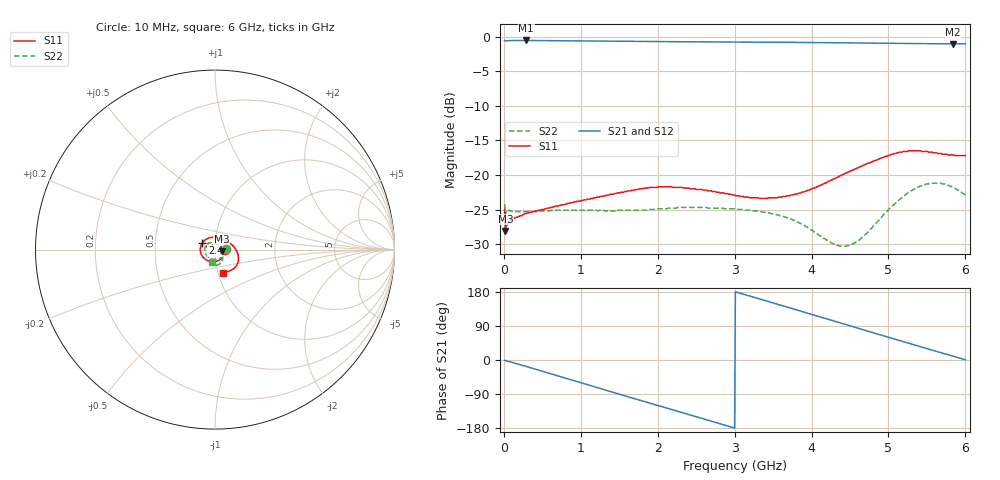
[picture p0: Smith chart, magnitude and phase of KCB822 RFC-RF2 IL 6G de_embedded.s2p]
!Agilent	"Technologies,N5230A,MY45001650,A.07.50.48"
!Agilent	N5230A:	A.07.50.48
!Date:	"Wednesday,"	February	"12,"	2014	15:18:42
!Correction:	S11(Full	2	"Port(1,2))"
!S21(Full	2	"Port(1,2))"
!S12(Full	2	"Port(1,2))"
!S22(Full	2	"Port(1,2))"
!S2P	File:	Measurements:	"S11,"	"S21,"	"S12,"	S22:
#	Hz	S	dB	R	50
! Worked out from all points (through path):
!   600 points, 10 MHz to 6 GHz, reference 50 ohm
!   highest |S21| = -0.55 dB at 290 MHz (marker M1); lowest = -1.0 dB at 5.84 GHz (marker M2)
!   group delay of S21, straight-line fit = 167 ps
!   lowest |S11| = -28.1 dB at 20 MHz (marker M3), VSWR 1.08, Z = 54 - j0.863 ohm
!   |S11| at or under -10 dB: start of sweep to end of sweep
!   |S22| runs from -30.3 to -21.2 dB; largest |S21 - S12| = 0.016
!   S11 on the Smith chart (normalised r, x): 10 MHz: 1.12, -0.00; 2.47 GHz: 0.87, +0.07; 6 GHz: 1.05, -0.28
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1e7  -25.00 -1.6  -0.55 -0.9  -0.55 -1.1  -24.20 3.1
2e7  -28.10 -11.7  -0.59 -1.4  -0.59 -1.4  -25.70 -4.1
5e7  -27.00 -6.7  -0.59 -3.4  -0.59 -3.4  -25.10 -4.4
2.9e8  -25.60 -18.8  -0.55 -16.9  -0.55 -17.0  -25.30 -13.0
6.4e8  -24.60 -46.1  -0.58 -38.2  -0.58 -38.2  -25.10 -33.7
1.01e9  -23.70 -79.3  -0.61 -60.5  -0.61 -60.5  -25.10 -59.7
1.26e9  -23.10 -103.0  -0.64 -75.6  -0.64 -75.6  -25.10 -79.6
1.51e9  -22.60 -126.0  -0.66 -90.6  -0.66 -90.6  -25.10 -101.0
1.77e9  -22.00 -149.0  -0.68 -106.0  -0.68 -106.0  -25.10 -123.0
2.01e9  -21.70 -170.0  -0.71 -121.0  -0.71 -121.0  -24.90 -142.0
2.47e9  -22.00 152.0  -0.74 -148.0  -0.74 -148.0  -24.70 -173.0
2.73e9  -22.40 131.0  -0.76 -163.0  -0.76 -163.0  -24.80 173.0
3.01e9  -23.00 109.0  -0.78 180.0  -0.78 180.0  -24.90 161.0
3.48e9  -23.30 71.3  -0.80 152.0  -0.80 152.0  -25.60 141.0
4.01e9  -22.00 35.4  -0.85 120.0  -0.85 120.0  -28.00 106.0
4.3e9  -20.50 19.4  -0.87 102.0  -0.87 102.0  -30.00 68.0
4.49e9  -19.50 9.1  -0.88 90.8  -0.88 90.8  -30.20 34.2
4.75e9  -18.30 -5.0  -0.92 75.0  -0.92 75.0  -28.00 -8.8
5.01e9  -17.20 -19.6  -0.95 59.2  -0.95 59.1  -24.90 -38.9
5.47e9  -16.60 -47.2  -1.02 31.5  -1.02 31.5  -21.40 -74.2
5.84e9  -17.10 -64.3  -1.04 10.1  -1.04 10.1  -21.80 -98.1
6e9  -17.20 -71.6  -1.03 0.6  -1.03 0.6  -22.90 -104.0
